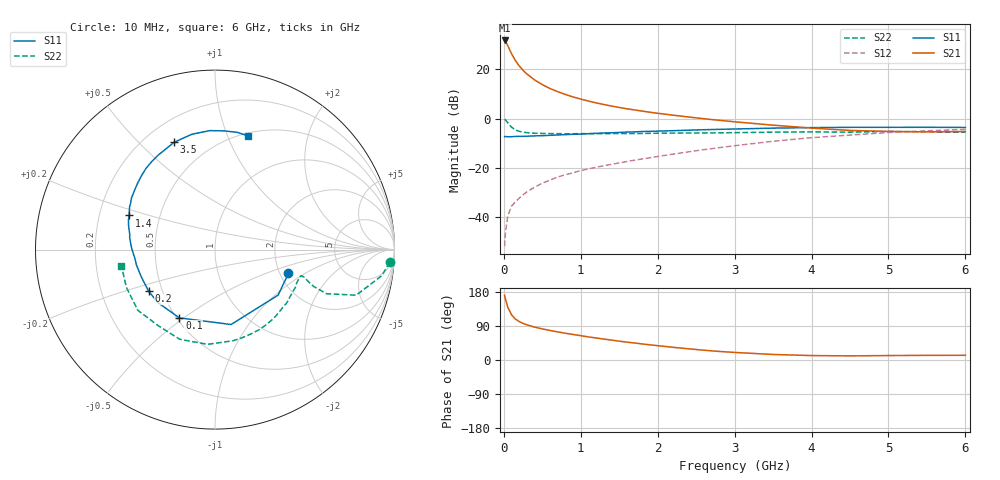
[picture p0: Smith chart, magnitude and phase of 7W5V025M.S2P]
! Infineon Technologies  Discrete & RF Semiconductors
! BFS17W
! Si NPN RF Bipolar Junction Transistor in SOT323
! VCE = 5 V  IC = 25 mA
! Common Emitter S-Parameters:  August  1999
# GHz  S  MA  R  50
!  f  S11  S21  S12  S22
! GHz  MAG  ANG  MAG  ANG  MAG  ANG  MAG  ANG
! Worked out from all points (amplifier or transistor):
!   36 points, 10 MHz to 6 GHz, reference 50 ohm
!   highest |S21| = 31.6 dB at 10 MHz (marker M1)
!   |S21| within 3 dB of that: start of sweep to 64.82 MHz
!   unconditionally stable (mu >= 1): 247 MHz to 2.112 GHz; 5.185 GHz to end of sweep
!   at 250 MHz: K = 1.01, MAG = 24.8 dB, |S12| = -30.9 dB
!   at 1.4 GHz: K = 1.16, MAG = 9.4 dB, |S12| = -18.6 dB
!   at 6 GHz: K = 1.05, MAG = -1.8 dB, |S12| = -4.4 dB
!   S11 on the Smith chart (normalised r, x): 10 MHz: 2.22, -0.72; 100 MHz: 0.52, -0.48; 200 MHz: 0.42, -0.24; 1.4 GHz: 0.33, +0.17; 3.5 GHz: 0.32, +0.64; 6 GHz: 0.53, +1.18
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0.01  0.4302 -18.0  38.17 170.8  0.0026 82.0  0.976 -4.1
0.02  0.4335 -35.8  37.07 161.7  0.0047 80.1  0.9406 -8.9
0.05  0.4269 -77.9  30.32 139.9  0.0106 67.4  0.8264 -17.9
0.1  0.429 -117.5  20.57 119.3  0.0168 60.5  0.6678 -21.6
0.15  0.4342 -137.2  14.97 108.1  0.0206 60.9  0.588 -20.5
0.2  0.4362 -147.9  11.65 101.4  0.0246 63.3  0.5512 -19.0
0.25  0.4357 -156.1  9.477 96.5  0.0285 65.3  0.5289 -17.7
0.3  0.4383 -160.9  7.975 92.8  0.0328 66.4  0.5181 -17.1
0.4  0.4458 -168.8  6.053 86.7  0.0408 68.1  0.5034 -16.8
0.5  0.4495 -174.0  4.866 82.1  0.049 69.7  0.4991 -17.2
0.6  0.4573 -178.0  4.058 77.9  0.0567 70.6  0.4956 -18.2
0.7  0.4654 178.6  3.503 74.2  0.0655 71.3  0.4939 -19.7
0.9  0.4799 172.0  2.739 67.4  0.0797 72.6  0.4917 -23.2
1.1  0.494 166.2  2.259 60.9  0.0957 72.7  0.4931 -27.4
1.4  0.5149 158.3  1.79 52.5  0.1181 73.3  0.4964 -34.5
1.8  0.5464 148.5  1.414 42.3  0.152 74.3  0.4989 -45.0
2.2  0.568 139.4  1.17 33.5  0.1903 74.0  0.5066 -55.9
2.8  0.604 125.7  0.921 22.6  0.2572 71.3  0.5141 -73.3
3.5  0.6397 110.9  0.734 14.6  0.3465 65.3  0.5294 -94.4
4.5  0.6636 92.6  0.574 10.9  0.463 52.3  0.529 -127.2
5.5  0.665 79.3  0.537 12.3  0.5646 39.1  0.5367 -156.9
6  0.6601 74.0  0.547 12.4  0.6042 32.7  0.5291 -170.0
